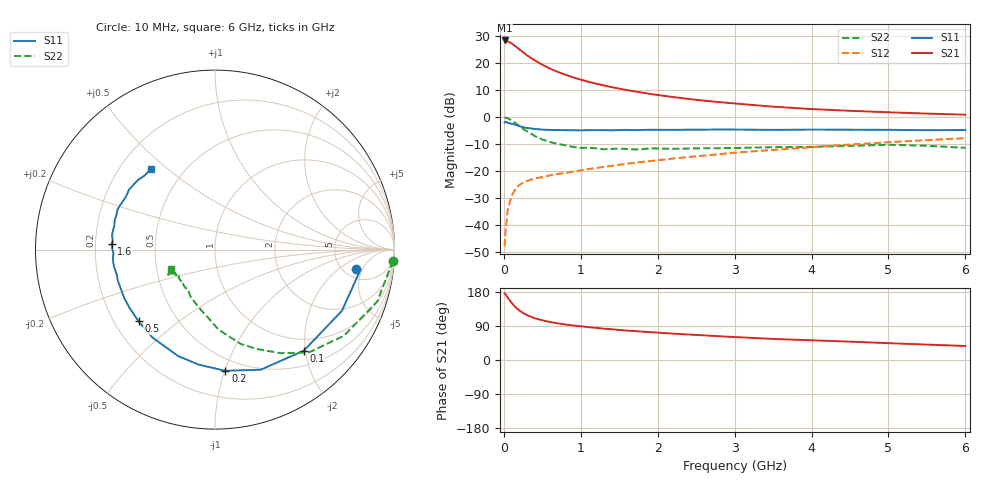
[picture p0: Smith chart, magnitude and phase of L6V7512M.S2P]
!  INFINEON TECHNOLOGIES Small Signal Semiconductors
! BFR380L3 , Si-NPN RF-Transistor in TSLP-3-1
!  Vce=0.75 V,  Ic=12.5 mA
! Common Emitter S-Parameters:  07. March 2005
#  GHz  S  MA  R  50
! f  S11  S21  S12  S22
! GHz  Mag  Ang  Mag  Ang  Mag  Ang  Mag  Ang
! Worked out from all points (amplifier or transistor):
!   36 points, 10 MHz to 6 GHz, reference 50 ohm
!   highest |S21| = 28.4 dB at 10 MHz (marker M1)
!   |S21| within 3 dB of that: start of sweep to 188.6 MHz
!   unconditionally stable (mu >= 1): 1.929 GHz to 5.336 GHz
!   at 250 MHz: K = 0.31, MSG = 24.2 dB, |S12| = -24.4 dB
!   at 1.4 GHz: K = 0.93, MSG = 14.6 dB, |S12| = -18.1 dB
!   at 6 GHz: K = 0.99, MSG = 4.3 dB, |S12| = -7.8 dB
!   S11 on the Smith chart (normalised r, x): 10 MHz: 6.44, -3.63; 100 MHz: 0.76, -1.97; 200 MHz: 0.40, -1.01; 500 MHz: 0.30, -0.36; 1.6 GHz: 0.27, +0.03; 6 GHz: 0.33, +0.44
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0.01  0.7901 -7.7  26.39 175.1  0.004 81.6  0.9953 -3.7
0.02  0.8186 -7.8  26.26 174.0  0.0069 86.8  0.9748 -7.4
0.05  0.7852 -25.7  25.5 164.6  0.0186 80.1  0.9495 -17.7
0.1  0.7498 -48.7  23.26 151.1  0.034 67.9  0.8643 -33.7
0.15  0.7159 -69.2  20.7 139.6  0.0463 59.1  0.7761 -47.6
0.2  0.6777 -85.1  18.12 130.9  0.0545 54.3  0.6844 -57.5
0.25  0.6476 -98.0  15.97 124.2  0.0602 49.6  0.6006 -67.2
0.3  0.6277 -109.1  14.05 118.6  0.0649 47.7  0.5452 -74.7
0.4  0.6012 -125.5  11.3 110.4  0.0721 44.9  0.4463 -87.5
0.5  0.5836 -136.9  9.363 104.8  0.0767 44.8  0.3825 -95.6
0.6  0.5764 -145.6  7.915 100.2  0.0824 44.8  0.3444 -103.3
0.8  0.5682 -157.8  6.09 93.7  0.092 47.4  0.2983 -116.7
0.9  0.5681 -162.8  5.435 91.2  0.0965 48.2  0.2786 -121.6
1.1  0.5693 -169.6  4.513 86.7  0.108 50.3  0.2694 -128.0
1.4  0.5661 -177.7  3.59 81.3  0.1238 53.0  0.2553 -135.7
1.6  0.5768 176.9  3.162 77.7  0.1358 54.0  0.255 -142.7
2.2  0.5768 166.6  2.347 69.6  0.1695 56.8  0.2563 -146.5
2.8  0.5869 157.7  1.891 62.8  0.204 58.5  0.2638 -151.9
3.5  0.5772 149.1  1.555 55.6  0.2447 57.8  0.2754 -151.5
4.5  0.5808 142.1  1.303 48.4  0.3077 57.4  0.2913 -151.5
5.5  0.5692 133.5  1.158 40.7  0.373 54.2  0.2926 -152.4
6  0.5737 128.3  1.104 37.0  0.4055 52.2  0.2678 -156.3
